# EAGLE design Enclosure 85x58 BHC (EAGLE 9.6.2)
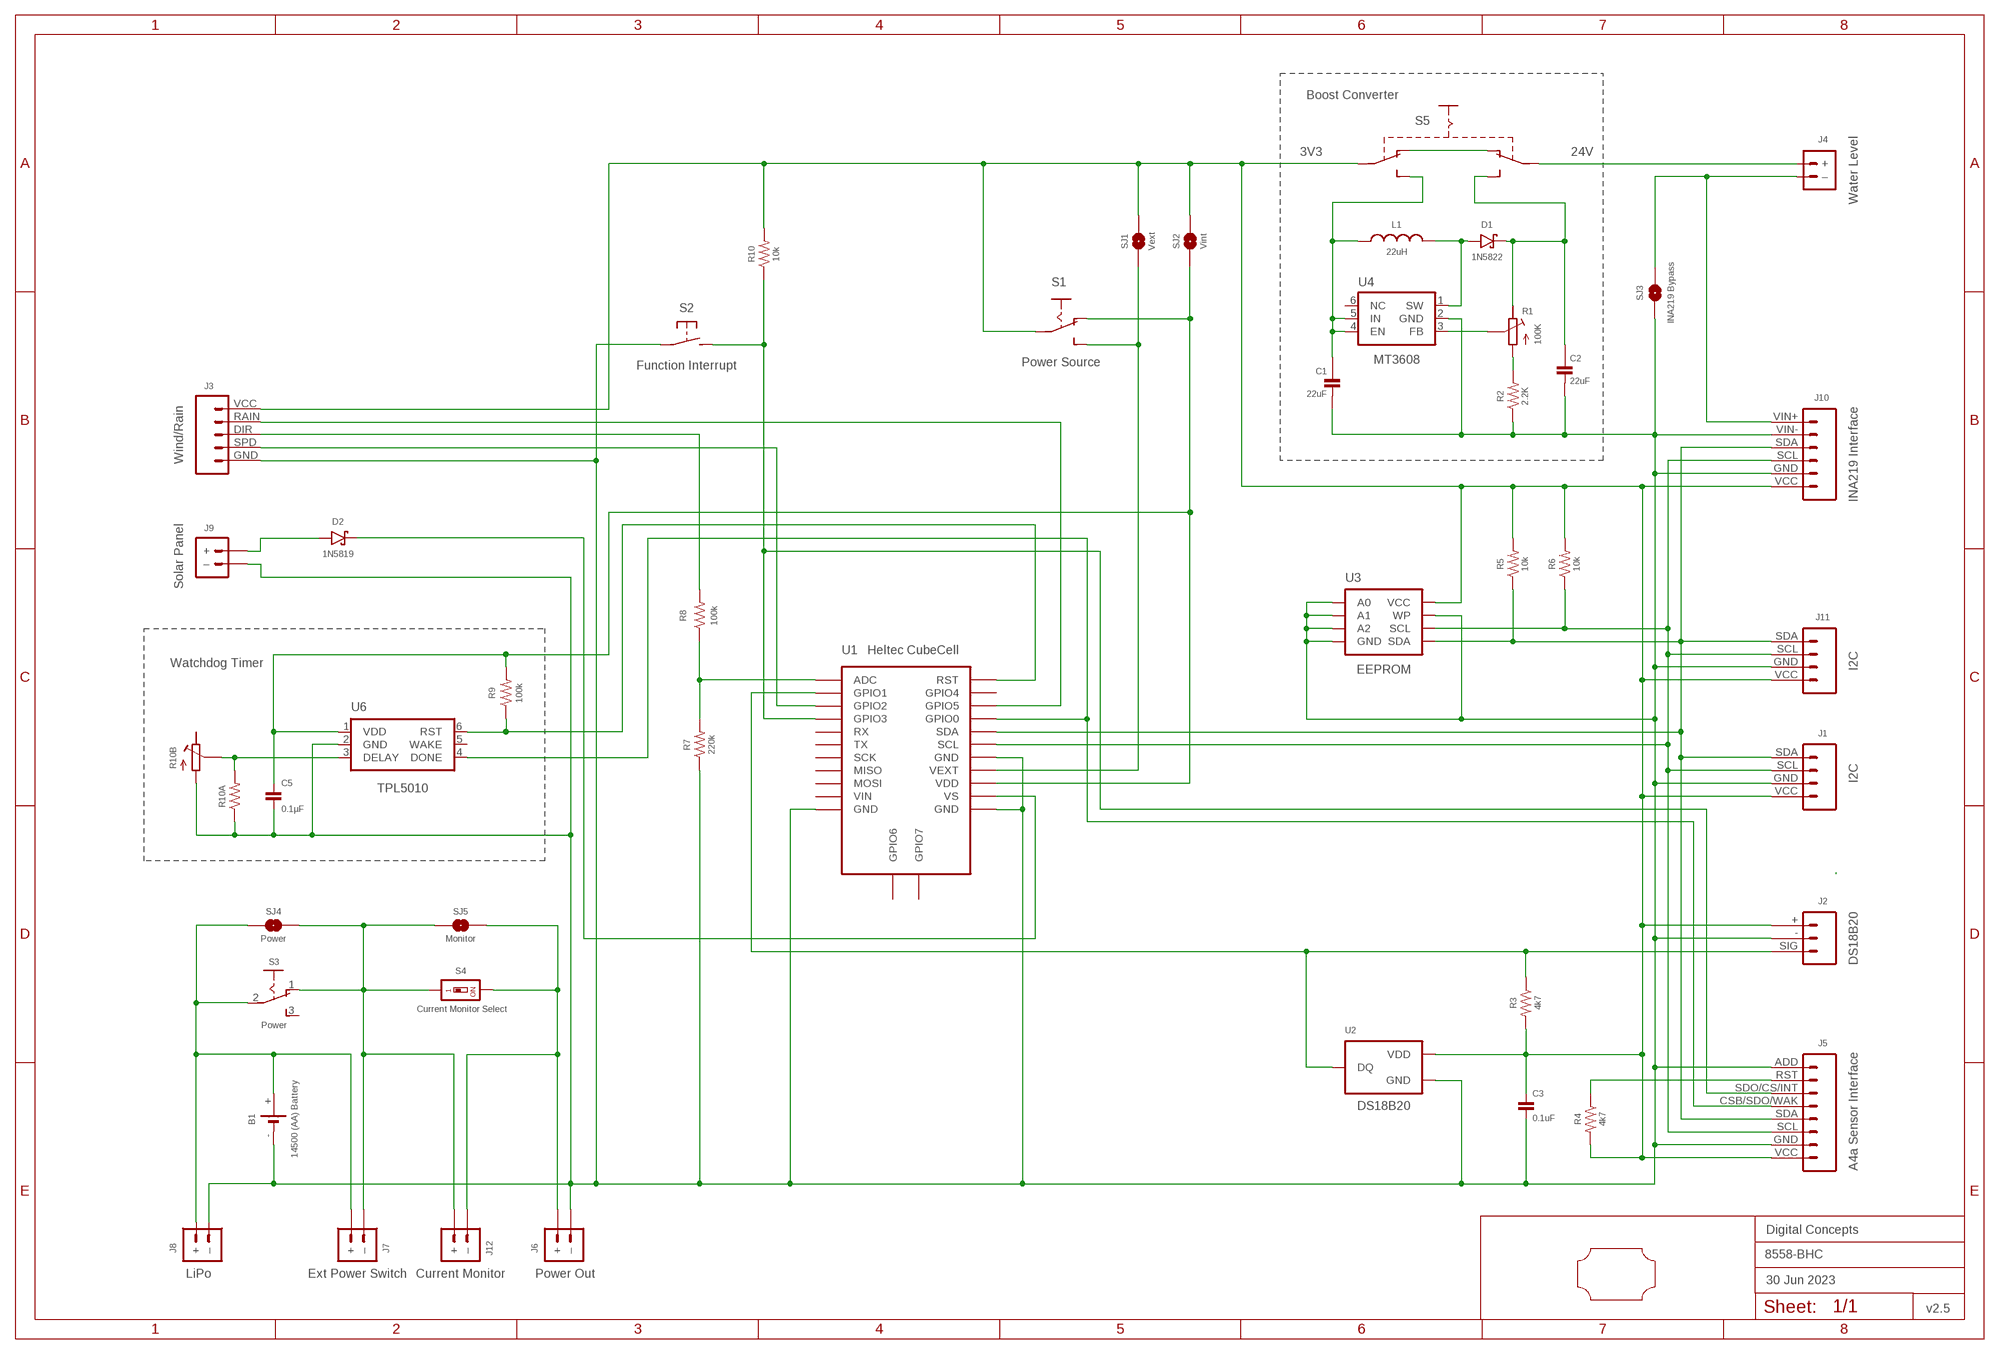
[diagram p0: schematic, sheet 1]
FRAME2 (A3L-LOC): DATE: 30 Jun 2023; OWNER: Digital Concepts; TITLE: 8558-BHC; VERSION: v2.5

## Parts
B1  14500 (AA) Battery  BATTERY-HOLDER-14500(AA)  [BATTERY-14500]
C1  22uF  CAPACITOR-1206  [C1206]
C2  22uF  CAPACITOR-1206  [C1206]
C3  0.1uF  CAPACITOR-0805  [C0805]
C5  0.1µF  CAPACITOR-0805  [C0805]
D1  1N5822  DIODE-SCHOTTKY-1N5822  [DIODE_SMB]
D2  1N5819  1N5819-SOD-123  [SOD-123]
J1  I2C  JST-PH2.0-4-VERTICAL-I2C  [JST-PH2.0-4-VERTICAL-I2C]
J2  DS18B20  JST-PH2.0-3-VERTICAL-DS18B20  [JST-PH2.0-3-VERTICAL]
J3  Wind/Rain  JST-PH2.0-5-VERTICAL-WEATHER  [JST-PH2.0-5-WEATHER]
J4  Water Level  JST-PH2.0-2-VERTICAL  [JST-PH2.0-2-VERTICAL=POWER]
J5  A4a Sensor Interface  HEADER-1X8-SENSOR  [CONN_08-SENSOR]
J6  Power Out  JST-GH1.25-2-HORIZONTAL-POWER  [JST-GH1.25-2-HORIZONTAL]
J7  Ext Power Switch  JST-PH2.0-2-DUAL-POWERJST-PTH-2  [JST-PH2.0-2-DUAL-POWER]
J8  LiPo  JST-PH2.0-2-MALE-HORIZONTALJST-PTH-2  [JST-PH2.0-2-HORIZONTAL]
J9  Solar Panel  JST-PH2.0-2-DUAL-POWERJST-PTH-2  [JST-PH2.0-2-DUAL-POWER]
J10  INA219 Interface  INA219-I2C-MODULE  [CONN_06-INA219]
J11  I2C  JST-PH2.0-4-HORIZONTAL-I2C  [JST-PH2.0-4-HORIZONTAL-I2C]
J12  Current Monitor  JST-PH2.0-2-HORIZONTAL-POWERJST-PTH-2  [JST-PH2.0-2-HORIZONTAL-POWER]
L1  22uH  INDUCTOR-CDRH104R/6D28L5038P  [CDRH104R+6D28]
R1  100K  RESISTOR-TRIMM-BAOTER-HORIZONTAL  [RTRIM64P]
R2  2.2K  RESISTORR0805  [R0805]
R3  4k7  RESISTORR0805  [R0805]
R4  4k7  RESISTORR0805  [R0805]
R5  10k  RESISTORR0805  [R0805]
R6  10k  RESISTORR0805  [R0805]
R7  220k  RESISTORR0805  [R0805]
R8  100k  RESISTORR0805  [R0805]
R9  100k  RESISTORR0805  [R0805]
R10  10k  RESISTORR0805  [R0805]
R10A  RESISTORR0805  [R0805]
R10B  RESISTOR-TRIMM-33  [RTRIM3*3]
S1  Power Source  SWITCH-SLIDE-SPDT-SMT  [SWITCH-SPDT-SMT]
S2  Function Interrupt  SWITCH-MOMENTARY-2-PIN  [SWITCH-2-PAD]
S3  Power  SWITCH-SLIDE-SPDT  [SWITCH-SLIDE-SPDT]
S4  Current Monitor Select  SWITCH-DIP-SWS001  [SMD-001]
S5  SWITCH-SLIDE-DPDT-PTH-S  [SWITCH-DPDT-PTH]
SJ1  Vext  SJ  [SJ]
SJ2  Vint  SJ-V-1  [SJ-VIA-1]
SJ3  INA219 Bypass  SJ  [SJ]
SJ4  Power  SJ  [SJ]
SJ5  Monitor  SJ  [SJ]
U1  Heltec CubeCell  HELTEC-CUBECELL  [HELTEC-CUBECELL]
U2  DS18B20  THERMOMETER-DS18B20  [TO-92]
U3  EEPROM  AT24CXX-EEPROM  [SOP-8]
U4  MT3608  [SOT-23-6@1]
U6  TPL5010  TPL5010DDCR  [SOT-23-6]
U$1  PCB-OUTLINE-C-85X58  [PROTO-28X18-OUTLINE-C]

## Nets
GND: B1.- C1.2 C2.2 C3.2 C5.2 J1.GND J2.- J3.GND J5.ADD J5.GND J6.-(–) J8.-(–) J9.-(–) J10.GND J10.VIN- J11.GND R2.1 R7.1 R10A.1 R10B.1(A) S2.P$1(P) SJ3.1 U1.GND@11(GND) U1.GND@14(GND) U1.GND@18(GND) U2.1(GND) U3.P$1(A0) U3.P$2(A1) U3.P$3(A2) U3.P$4(GND) U3.P$7(WP) U4.2(GND) U6.2(GND)
N$1: D2.A J9.+
N$2: J3.DIR R8.2
N$4: B1.+ J7.+ J8.+ S3.2(P) SJ4.2
N$5: D2.C U1.VS
N$6: D1.A L1.1 U4.1(SW)
N$7: C5.1 R9.2 S1.P$1(O) SJ2.2 U1.VDD U6.1(VDD)
N$8: J1.SCL J5.SCL J10.SCL J11.SCL R6.1 U1.SCL U3.P$6(SCL)
N$9: J5.RST R4.1
N$10: R7.2 R8.1 U1.ADC
N$11: J1.SDA J5.SDA J10.SDA J11.SDA R5.1 U1.SDA U3.P$5(SDA)
N$12: J3.SPD U1.GPIO2
N$14: J6.+ J12.-(–) S4.2 SJ5.1
N$15: J4.-(–) J10.VIN+ SJ3.2
N$18: J2.SIG R3.1 U1.GPIO1 U2.2(DQ)
N$19: J5.SDO/CS/INT R10.1 S2.P$2(S) U1.GPIO3
N$20: C2.1 D1.C R1.3(E) S5.P$3(S1)
N$21: S1.P$2(S) SJ1.2 U1.VEXT
N$22: J3.RAIN U1.GPIO5
N$23: R1.1(A) R2.2
N$24: R1.2(S) U4.3(FB)
N$25: C1.1 L1.2 S5.P$6(S2) U4.4(EN) U4.5(IN)
N$26: S5.P$1(O1) S5.P$4(O2)
N$27: J4.+ S5.P$2(P1)
N$28: J5.CSB/SDO/WAK U1.GPIO0 U6.4(DONE)
N$36: R10A.2 R10B.2(S) U6.3(DELAY)
N$37: R9.1 U1.RST U6.6(RST)
N$39: J7.-(–) J12.+ S3.1(O) S4.1 SJ4.1 SJ5.2
VCC: C3.1 J1.VCC J2.+ J3.VCC J5.VCC J10.VCC J11.VCC R3.2 R4.2 R5.2 R6.2 R10.2 S1.COMMON(P) S5.P$5(P2) SJ1.1 SJ2.1 SJ2.1@V U2.3(VDD) U3.P$8(VCC)
Unconnected: R10B.3(E) S3.3(S) U1.GPIO4 U1.GPIO6 U1.GPIO7 U1.MISO U1.MOSI U1.RX U1.SCK U1.TX U1.VIN U4.6(NC) U6.5(WAKE)

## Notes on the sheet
- Boost Converter
- 3V3 | 24V
- Watchdog Timer

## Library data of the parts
B1 = digitalconcepts:BATTERY-HOLDER-14500(AA): 14500 (AA) battery holder
C1 C2 = digitalconcepts:CAPACITOR-1206: 1206 Capacitor
C3 C5 = digitalconcepts:CAPACITOR-0805: 0805 Capacitor
D1 = digitalconcepts:DIODE-SCHOTTKY-1N5822: 1N5822 Schottky Diode SMB
D2 = digitalconcepts:1N5819-SOD-123: 1N5819 Schottky Diode SOD-123
J1 = digitalconcepts:JST-PH2.0-4-VERTICAL-I2C: PH2.0 4P I2C Vertical Connector
J2 = digitalconcepts:JST-PH2.0-3-VERTICAL-DS18B20: DS18B20 PH2.0 Vertical PCB Connector
J3 = digitalconcepts:JST-PH2.0-5-VERTICAL-WEATHER: PH2.0 5P Vertical Weather Connector
J4 = digitalconcepts:JST-PH2.0-2-VERTICAL: PH2.0 2P PCB Connector
J5 = digitalconcepts:HEADER-1X8-SENSOR: IoT Sensors 1x8 Pin Header for 'Sandwich' IoT Sensors
J6 = digitalconcepts:JST-GH1.25-2-HORIZONTAL-POWER: JST GH1.25 2P PTH Connector (Power)
J7 J9 = digitalconcepts:JST-PH2.0-2-DUAL-POWER: JST PH2.0 2P PTH Dual-Side Connector (Power); PROD_ID: CONN-09863; SKU: PRT-09914
J8 = digitalconcepts:JST-PH2.0-2-MALE-HORIZONTAL: PH2.0 2P Right Angle PCB Connector; PROD_ID: CONN-09863; SKU: PRT-09914
J10 = digitalconcepts:INA219-I2C-MODULE: INA219 I2C Module
J11 = digitalconcepts:JST-PH2.0-4-HORIZONTAL-I2C: PH2.0 4P I2C Horizontal Connector
J12 = digitalconcepts:JST-PH2.0-2-HORIZONTAL-POWER: PH2.0 2P Right Angle PCB Connector; PROD_ID: CONN-09863; SKU: PRT-09914
L1 = digitalconcepts:INDUCTOR-CDRH104R/6D28: Inductor; SPICEPREFIX: L
R1 = digitalconcepts:RESISTOR-TRIMM-BAOTER-HORIZONTAL: Trimm Resistor - Horizontal BAOTER
R2-R10 R10A = digitalconcepts:RESISTOR: Resistor; SPICEPREFIX: R
R10B = digitalconcepts:RESISTOR-TRIMM-3*3: Trimm Resistor - 3*3 SMD
S1 = digitalconcepts:SWITCH-SLIDE-SPDT-SMT: Mini Sliding Switch SPDT SMT
S2 = digitalconcepts:SWITCH-MOMENTARY-2-PIN: 2 Pin Momentary Switch
S3 = digitalconcepts:SWITCH-SLIDE-SPDT: Mini Sliding Switch SPDT
S4 = digitalconcepts:SWITCH-DIP-SWS001: SMD Dip Switch 1 pol.
S5 = digitalconcepts:SWITCH-SLIDE-DPDT-PTH-S: Switch DPDT PTH-S
SJ1 SJ3-SJ5 = digitalconcepts:SJ: Solder Jumper
SJ2 = digitalconcepts:SJ-V-1: Solder Jumper with single Pad Via
U1 = digitalconcepts:HELTEC-CUBECELL: Heltec CubeCell Development Board
U2 = digitalconcepts:THERMOMETER-DS18B20: Digital Thermometer -55C-125C TO92-3; AVAILABILITY: Bad; DESCRIPTION: Temperature Sensor Digital, Local -55°C ~ 125°C 12 b 8-uMAX; MF: Maxim Integrated; MP: DS18B20; PACKAGE: TO-92 Maxim Integrated; PRICE: None
U3 = digitalconcepts:AT24CXX-EEPROM: AT24Cxx EEPROM SOP-8
U4 = digitalconcepts:MT3608: MT3608 DC-DC Step-Up Voltage Converter
U6 = digitalconcepts:TPL5010DDCR: TPL5010 Nano-Power System Timer with Watchdog
U$1 = digitalconcepts:PCB-OUTLINE-C-85X58: PCB outline with cut-out for 85 x 58 enclosure

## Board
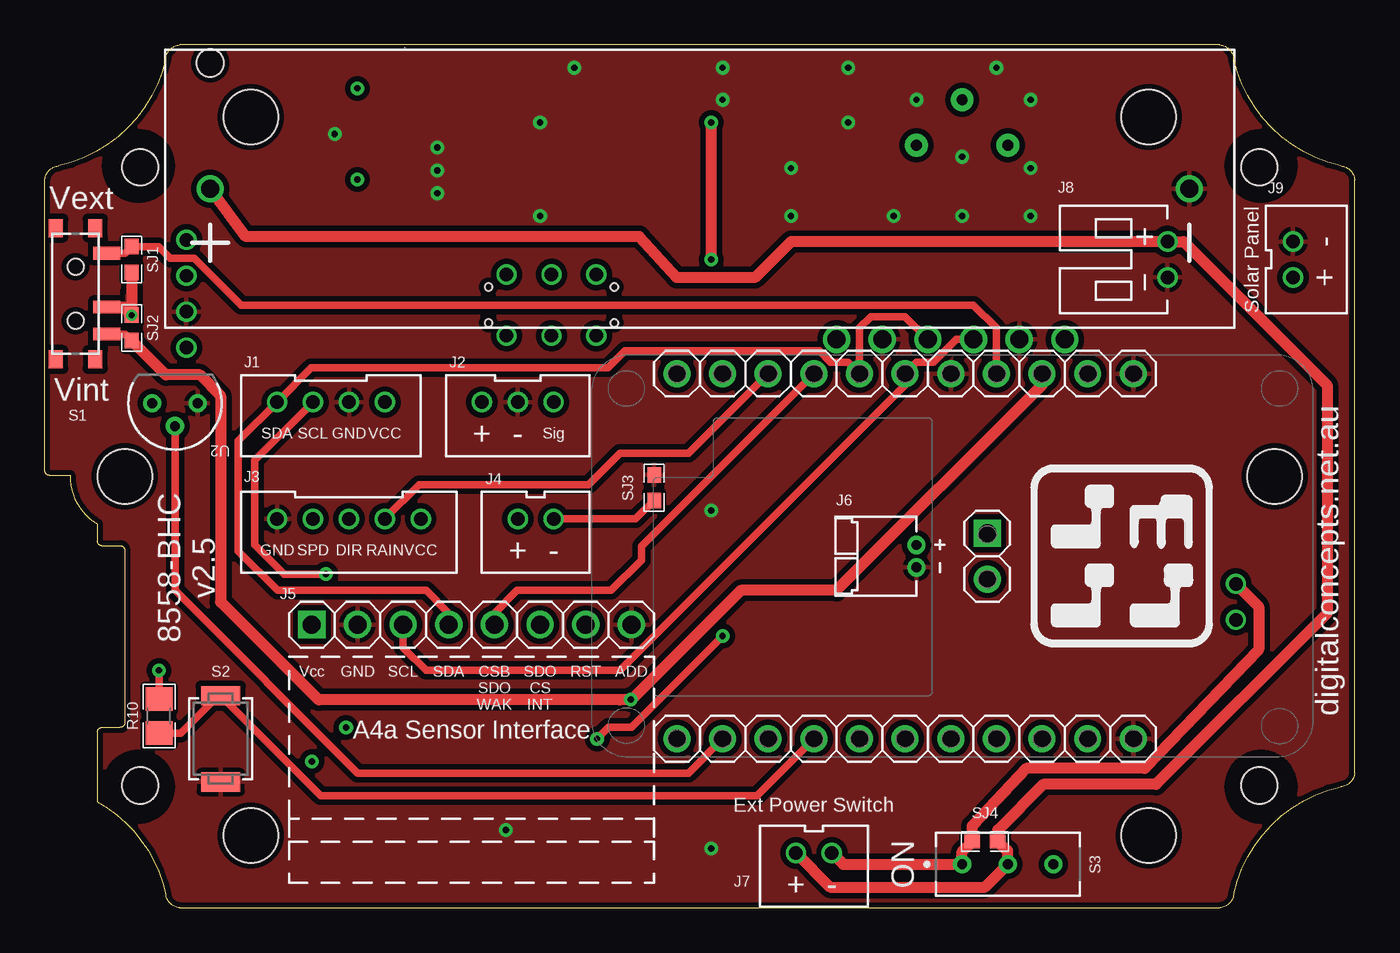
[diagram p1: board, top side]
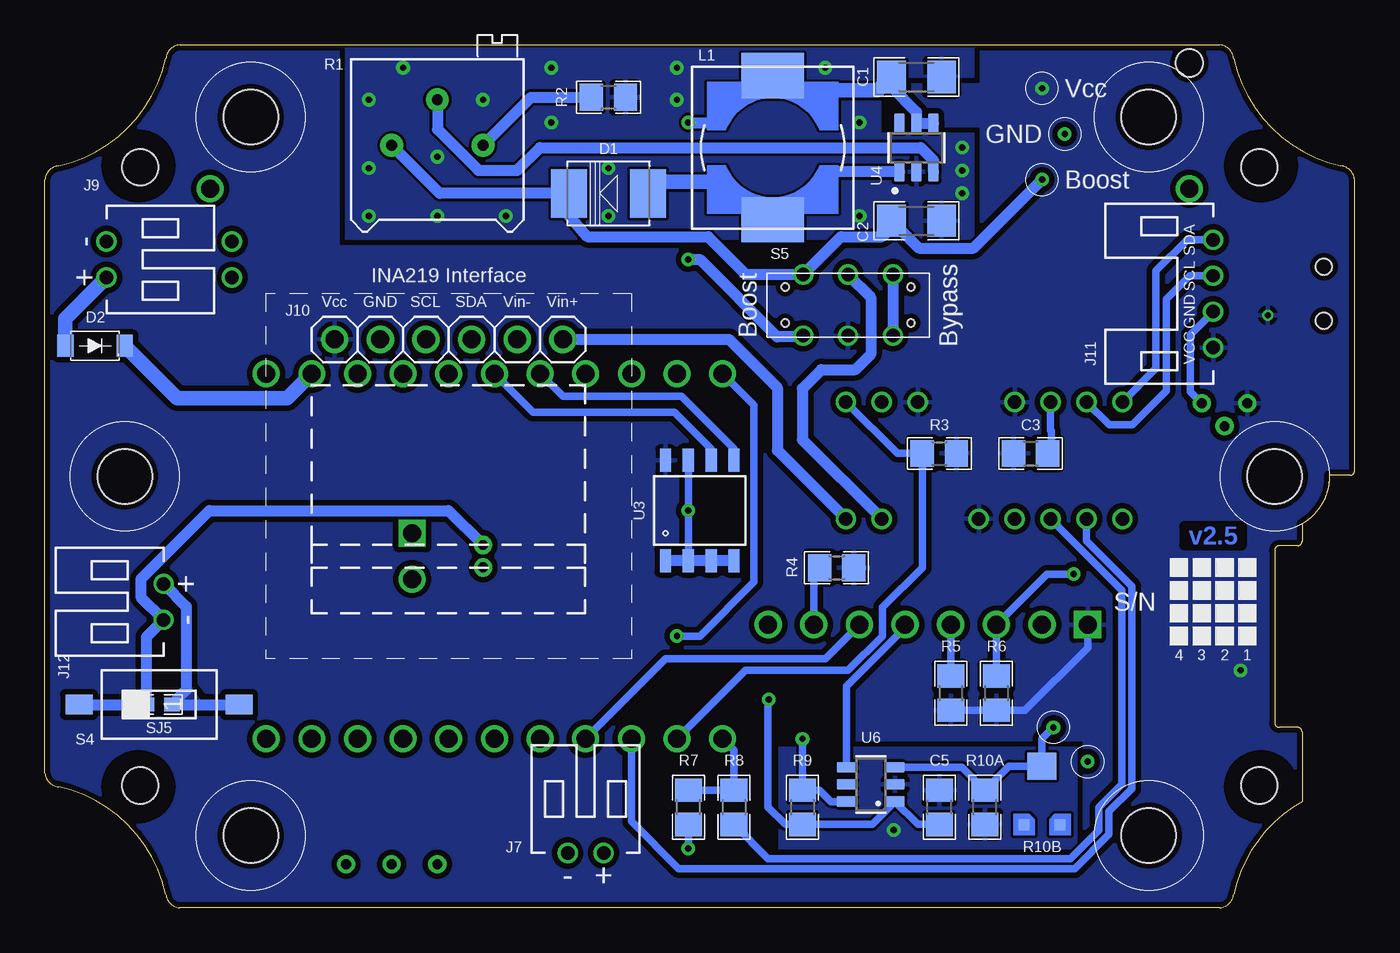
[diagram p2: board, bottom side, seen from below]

Size 72.9 x 48.01 mm. Coordinates in mm from the lower left corner, seen from the top.
Copper layers (1*16): Top 0.035mm / dielectric 1.5mm / Bottom 0.035mm
Design rules "default *": minimum track width 6mil, minimum drill 0.35mm, track to track 6mil, track to pad 6mil, pad to pad 6mil, via to via 6mil, smd to smd 6mil, copper to edge 6mil, drill to drill 6mil, minimum pad ring 1mil, minimum via ring 8mil, stop-mask expansion 4mil, vias tented up to drill 0mil, thermal gap 10mil

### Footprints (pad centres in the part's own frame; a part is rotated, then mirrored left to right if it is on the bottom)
BATTERY-14500 = drill 1: + -27.25,0; - 27.25,0 | hole 1.524: -27.25,7
C1206 = smd 1.6 x 1.8: 1 -1.4,0; 2 1.4,0
C0805 = smd 1.3 x 1.5: 1 -0.95,0; 2 0.95,0
DIODE_SMB = smd 2 x 2.7: A 2.2,0; C -2.2,0
SOD-123 = smd 0.91 x 1.22: A -1.65,0; C 1.65,0
JST-PH2.0-4-VERTICAL-I2C = drill 0.75: GND 1,0; SCL -1,0; SDA -3,0; VCC 3,0
JST-PH2.0-3-VERTICAL = drill 0.75: + -2,0; - 0,0; SIG 2,0
JST-PH2.0-5-WEATHER = drill 0.75: DIR 0,0; GND 4,0; RAIN -2,0; SPD 2,0; VCC -4,0
JST-PH2.0-2-VERTICAL=POWER = drill 0.75: + -1,0; - 1,0
CONN_08-SENSOR = drill 1 pad 1.524: ADD 17.78,0; CSB/SDO/WAK 10.16,0; GND 2.54,0; RST 15.24,0; SCL 5.08,0; SDA 7.62,0; SDO/CS/INT 12.7,0 | drill 1 pad 1.524 square: VCC 0,0
JST-GH1.25-2-HORIZONTAL = drill 0.55 pad 1.016: + -0.625,0; - 0.625,0
JST-PH2.0-2-DUAL-POWER = drill 0.75: + 1,0; - -1,0
JST-PH2.0-2-HORIZONTAL = drill 0.75: + 1,0; - -1,0
CONN_06-INA219 = drill 1 pad 1.524: GND 2.54,0; SCL 5.08,0; SDA 7.62,0; VCC 0,0; VIN+ 12.7,0; VIN- 10.16,0
JST-PH2.0-4-HORIZONTAL-I2C = drill 0.75: GND -1,0; SCL 1,0; SDA 3,0; VCC -3,0
JST-PH2.0-2-HORIZONTAL-POWER = drill 0.75: + 1,0; - -1,0
CDRH104R+6D28 = smd 2.5 x 3.5: 1 -4,0; 2 4,0
RTRIM64P = drill 0.61 pad 1.27: 1 0,-2.54; 2 2.54,0; 3 0,2.54
R0805 = smd 1.3 x 1.5: 1 -0.95,0; 2 0.95,0
RTRIM3*3 = smd 0.6 x 0.6: 1 -1,-1.6; 3 1,-1.6 | smd 1.6 x 1.5: 2 0,1.65
SWITCH-SPDT-SMT = smd 0.7 x 1.5: COMMON 0.75,1.75; P$1 2.25,1.75; P$2 -2.25,1.75 | smd 1 x 0.8: GND@1 3.65,-1.1; GND@2 3.65,1.1; GND@3 -3.65,1.1; GND@4 -3.65,-1.1 | hole 0.9: -1.5,0; 1.5,0
SWITCH-2-PAD = smd 1.067 x 2.184: P$1 -2.4,0; P$2 2.4,0
SWITCH-SLIDE-SPDT = drill 0.55 pad 1.016: 1 -2.54,0; 2 0,0; 3 2.54,0
SMD-001 = smd 1.1 x 1.5: 1 0,-4.45; 2 0,4.45
SWITCH-DPDT-PTH = drill 0.75: P$1 -1.7,2.5; P$2 -1.7,0; P$3 -1.7,-2.5; P$4 1.7,2.5; P$5 1.7,0; P$6 1.7,-2.5 | hole 0.42: 1,3.5; -1,3.5; 1,-3.5; -1,-3.5
SJ = smd 0.864 x 0.762: 1 -0.711,0; 2 0.711,0
SJ-VIA-1 = smd 0.864 x 0.762: 1 -0.711,0; 2 0.711,0 | drill 0.35 pad 0.61: 1@V -0.711,0
HELTEC-CUBECELL = drill 1: ADC 0,0; GND@11 0,25.4; GND@14 -20.32,25.4; GND@18 -20.32,15.24; GPIO0 -20.32,7.62; GPIO1 0,2.54; GPIO2 0,5.08; GPIO3 0,7.62; GPIO4 -20.32,2.54; GPIO5 -20.32,5.08; GPIO6 -8.89,17.272; MISO 0,17.78; MOSI 0,20.32; RST -20.32,0; RX 0,10.16; SCK 0,15.24; SCL -20.32,12.7; SDA -20.32,10.16; TX 0,12.7; VDD -20.32,20.32; VEXT -20.32,17.78; VIN 0,22.86; VS -20.32,22.86 | drill 1 square: GPIO7 -11.43,17.272
TO-92 = drill 0.55 pad 1.016: 1 -1.27,0; 2 0,1.27; 3 1.27,0
SOP-8 = smd 0.635 x 1.27: P$1 -1.905,-2.794; P$2 -0.635,-2.794; P$3 0.635,-2.794; P$4 1.905,-2.794; P$5 1.905,2.794; P$6 0.635,2.794; P$7 -0.635,2.794; P$8 -1.905,2.794
SOT-23-6@1 = smd 1.1 x 0.6: 1 -1.35,0.95; 2 -1.35,0; 3 -1.35,-0.95; 4 1.35,-0.95; 5 1.35,0; 6 1.35,0.95
SOT-23-6 = smd 1.1 x 0.6: 1 -1.35,0.95; 2 -1.35,0; 3 -1.35,-0.95; 4 1.35,-0.95; 5 1.35,0; 6 1.35,0.95
PROTO-28X18-OUTLINE-C = hole 2.032: -31.14,17.196; -31.14,-17.196; 31.14,-17.196; 31.14,17.196 | hole 3.048: -24.994,19.99; -32.004,0; -24.994,-19.99; 24.994,-19.99; 32.004,0; 24.994,19.99

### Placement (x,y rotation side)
B1  36.45,40.01 0 top
C1  24.38,46.23 0 bottom
C2  24.38,38.23 0 bottom
C3  18.03,25.27 0 bottom
C5  23.11,5.59 90 bottom
D1  41.53,39.75 0 bottom
D2  70.1,31.27 0 bottom
J1  15.92,28.13 0 top
J2  26.32,28.13 0 top
J3  16.92,21.63 180 top
J4  27.32,21.63 0 top
J5  14.86,15.75 0 top
J6  48.51,19.56 270 top
J7  42.8,3.05 0 bottom
J8  62.48,36.07 90 top
J9  69.47,36.07 270 bottom
J10  56.77,31.62 0 bottom
J11  7.87,34.16 90 bottom
J12  66.29,17.02 90 bottom
L1  32.38,42.29 90 bottom
R1  51.05,42.42 90 bottom
R2  41.53,45.09 180 bottom
R3  23.11,25.27 0 bottom
R4  28.83,18.92 0 bottom
R5  22.48,11.94 270 bottom
R6  19.94,11.94 270 bottom
R7  37.08,5.59 90 bottom
R8  34.54,5.59 270 bottom
R9  30.73,5.59 270 bottom
R10  6.35,10.67 90 top
R10A  20.57,5.59 90 bottom
R10B  17.4,6.22 0 bottom
S1  1.7,34.16 270 top
S2  9.78,9.4 90 top
S3  53.59,2.41 0 top
S4  66.55,11.3 90 bottom
S5  28.19,33.53 270 bottom
SJ1  4.83,36.07 90 top
SJ2  4.83,32.26 270 top
SJ3  33.91,23.37 270 top
SJ4  52.32,3.68 0 top
SJ5  66.55,11.3 0 bottom
U1  35.18,9.4 270 top
U2  7.24,28.07 180 top
U3  36.45,22.1 0 bottom
U4  24.38,42.29 90 bottom
U6  26.92,6.86 180 bottom
U$1  36.45,24 0 top

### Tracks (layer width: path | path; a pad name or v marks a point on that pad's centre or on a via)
$X1
  cutout Bottom: 67.69,43.31 arc180 67.69,39.24 arc180
$X2
  cutout Bottom: 67.69,8.76 arc180 67.69,4.7 arc180
$X3
  cutout Bottom: 5.21,8.76 arc180 5.21,4.7 arc180
$X4
  cutout Bottom: 5.21,43.31 arc180 5.21,39.24 arc180
$X5
  cutout Top: 5.21,43.31 arc180 5.21,39.24 arc180
$X6
  cutout Top: 67.69,43.31 arc180 67.69,39.24 arc180
$X7
  cutout Top: 67.69,8.76 arc180 67.69,4.7 arc180
$X8
  cutout Top: 5.21,8.76 arc180 5.21,4.7 arc180
GND  (via drill 0.35)
  Bottom 0.406: C3.2 16.89,25.47 16.89,26.54 16.92,26.57 J1.GND | R7.1 v37.08,3.3 | U3.P$7 v37.08,22.1 U3.P$2 | J11.GND 9.14,31.89 9.14,28.7 U2.1
  Bottom 0.61: U3.P$4 U3.P$3 U3.P$2 U3.P$1
  other vias: 21.84,42.29 27.56,43.69 37.72,44.96 37.72,46.74 44.7,46.74 44.7,43.69 41.53,38.48 47.24,38.48 51.05,38.48 51.05,41.78 54.86,38.48 54.86,41.15 52.96,46.74 21.84,39.75 48.51,44.96 54.86,44.96 27.56,38.48 41.53,41.15 16.13,43.05 21.84,41.02 29.46,46.74 25.65,4.32
  pour Top (isolate 0.305, rank 2): -2.08,49.93 -2.08,-1.97 74.92,-1.97 74.92,49.93
  pour Bottom (rank 2): 21.21,48.13 21.21,46.23 26.42,46.23 26.42,43.05 21.21,43.05 21.21,37.21 56.13,37.21 56.13,48.13
  pour Bottom: 32,8.89 15.49,8.89 15.49,3.3 32,3.3
GND1  (via drill 0.35)
  other vias: 14.86,8.13
N$1
  Bottom 0.813: J9.+ 71.75,32.78 D2.A
N$2
  Bottom 0.406: J3.DIR 12.95,17.67 12.95,6.86 14.22,5.59 14.22,4.32 15.81,2.73 32.64,2.73 R8.2
N$4
  Top 0.61: B1.+ 11.18,37.34 33.09,37.34 35.18,35.05 39.51,35.05 41.53,37.07 J8.+ 63.39,37.07 71.37,29.08 71.37,16.38 61.85,6.86 55.58,6.86 53.03,4.32 SJ4.2 53.52,3.19 53.59,3.18 S3.2 52.32,1.14 43.7,1.14 J7.+
N$5
  Bottom 0.813: D2.C 65.53,28.35 59.41,28.35 U1.VS
N$6
  Bottom 0.61: L1.1 31.75,38.29 29.1,40.94 U4.1
  Bottom 0.813: D1.A 38.69,40.39 35.17,40.39 33.08,38.29 L1.1
N$7  (via drill 0.35)
  Top 0.406: SJ2.2 4.46,31.91 S1.P$1
  Top 0.61: 32.59,11.56 32.64,11.56 38.73,17.65 44.07,17.65 55.5,29.08 U1.VDD | SJ2.2 6.73,29.64 8.64,29.64 9.78,28.5 9.78,17.02 15.24,11.56 32,11.56 32.59,11.56 | v32.61,11.58 32.59,11.56
  Bottom 0.406: C5.1 24.3,4.64 U6.1 26.84,4.64 R9.2 31.69,4.64 32.64,5.59 32.64,11.56 v32.61,11.58
N$8  (via drill 0.35)
  Top 0.406: J5.SCL 19.94,14.48 21.21,13.21 32,13.21 47.88,29.08 U1.SCL 48.51,30.35 49.47,30.35 50.74,31.62 J10.SCL | v15.64,18.57 13.31,18.57 11.68,20.19 11.68,24.9 J1.SCL
  Bottom 0.406: v15.64,18.57 17.12,18.57 J5.SCL R6.1 | U3.P$6 35.81,25.53 37.85,27.56 45.72,27.56 U1.SCL | J11.SCL 9.16,35.16 10.47,33.85 10.47,28.77 12.38,26.86 13.65,26.86 J1.SCL
N$9
  Bottom 0.406: R4.1 30.1,18.6 J5.RST
N$10
  Bottom 0.406: R7.2 R8.1 34.54,8.76 U1.ADC
N$11
  Top 0.406: J10.SDA 47.88,32.89 45.97,32.89 45.34,32.26 U1.SDA 44.7,30.35 43.74,30.35 43.1,30.99 32.28,30.99 31.33,30.04 14.82,30.04 J1.SDA 10.77,25.98 10.77,19.84 12.95,17.65 21.21,17.65 22.48,16.38 J5.SDA
  Bottom 0.406: J11.SDA 9.32,37.16 11.05,35.43 11.05,30 J1.SDA | U1.SDA 44.07,28.45 37.46,28.45 34.54,25.53 U3.P$5 | J5.SDA R5.1
N$12
  Bottom 0.406: J3.SPD 14.92,20.42 12.39,17.9 12.39,6.63 13.66,5.36 13.66,4.09 15.58,2.17 37.63,2.17 40.26,4.8 U1.GPIO2
N$14
  Bottom 0.61: S4.2 SJ5.1 67.26,15.05 J12.- 67.56,17.29 67.56,18.29 63.75,22.1 50.43,22.1 J6.+
N$15
  Top 0.406: J4.- 32.88,21.63 SJ3.2
  Bottom 0.61: J4.- 32.13,25.44 32.13,28.94 34.81,31.62 J10.VIN+
N$18
  Top 0.406: U1.GPIO1 35.81,7.49 17.4,7.49 7.24,17.65 U2.2
  Bottom 0.406: J2.SIG 25.46,25.27 R3.1 24.06,18.93 26.29,16.71 26.29,15.11 28.19,13.21 33.91,13.21 U1.GPIO1
N$19
  Top 0.406: R10.1 7.56,9.72 9.64,11.8 S2.P$2 15.35,6.22 39.62,6.22 U1.GPIO3
  Bottom 0.406: U1.GPIO3 38.35,13.84 29.46,13.84 J5.SDO/CS/INT
N$20  (via drill 0.35)
  Bottom 0.61: v17.4,40.51 21.21,36.7 24.26,36.7 C2.1 25.78,37.84 26.29,37.34 28.58,37.34 S5.P$3 33.87,35.23 35.98,37.34 42.71,37.34 43.73,38.51 D1.C 50.93,39.75 R1.3
N$21
  Top 0.406: U1.VEXT 52.96,32.26 51.69,33.53 10.92,33.53 8.31,36.14 6.96,36.14 6.34,36.78 SJ1.2 4.46,36.41 S1.P$2
N$22
  Top 0.406: J3.RAIN 20.82,23.54 30.27,23.54 32,25.27 35.81,25.27 U1.GPIO5
N$23
  Bottom 0.61: R1.1 45.85,45.09 R2.2
N$24
  Bottom 0.61: R1.2 51.05,43.31 48.77,41.02 46.61,41.02 45.34,42.29 24.15,42.29 23.43,41.58 U4.3
N$25  (via drill 0.35)
  Top 0.61: v37.08,43.69 v37.08,36.07
  Bottom 0.61: C1.1 25.78,45.67 24.38,44.27 U4.5 U4.4 | v37.08,43.69 35.81,43.69 33.21,46.29 L1.2 | 30.69,31.76 32.14,31.76 36.45,36.07 v37.08,36.07
  Bottom 0.813: C1.1 26.53,45.48 31.58,45.48 L1.2 | S5.P$6 30.69,31.76
N$26
  Bottom 0.61: S5.P$1 S5.P$4
N$27
  Bottom 0.61: J4.+ 30.73,26.05 30.73,28.88 29.68,29.93 27.77,29.93 26.92,30.78 26.92,33.96 S5.P$2
N$28
  Top 0.406: U1.GPIO0 33.2,20.12 33.2,19.33 31.52,17.65 26.29,17.65 25.02,16.38 J5.CSB/SDO/WAK
  Bottom 0.406: J5.CSB/SDO/WAK 25.02,15.59 28.27,12.33 U6.4
N$36  (via drill 0.35)
  Bottom 0.406: U6.3 21.84,7.81 R10A.2 19.24,7.87 R10B.2 17.4,9.4 v16.76,10.03
N$37  (via drill 0.35)
  Top 0.406: v30.73,9.4 31.37,10.03 32.64,10.03 v37.72,15.11
  Bottom 0.406: U6.6 29.15,5.91 29.78,6.54 R9.1 v30.73,9.4 | U1.RST 33.42,27.96 33.42,18.14 36.45,15.11 v37.72,15.11
N$39
  Top 0.61: J12.+ 67.56,16.75 67.56,14.35 61.21,7.75 54.62,7.75 51.61,4.55 SJ4.1 51.05,3.12 S3.1 44.43,2.41 J7.-
  Bottom 0.61: J12.+ 65.02,16.75 65.02,12.12 SJ5.2 S4.1
  pour Bottom: 65.85,11.3 65.02,12.12 64.39,11.3
VCC  (via drill 0.35)
  Top 0.406: R10.2 v6.35,13.21
  Top 0.61: S1.COMMON 4.38,33.41 SJ2.1@V SJ1.1
  Bottom 0.406: R5.2 R6.2 18.35,10.99 14.86,14.48 J5.VCC
  other vias: 17.4,45.59
  pour Bottom (isolate 0.305, rank 5): -1.08,48.93 -1.08,-0.97 73.92,-0.97 73.92,48.93
  pour Top: 4.22,33.46 4.7,33.93 4.7,32.98

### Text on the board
Bottom: v2.5
tPlace: digitalconcepts.net.au | 8558-BHC / v2.5
bPlace: Vin+ | Vin- | SDA | SCL | GND | Vcc | S/N | 1 | 2 | 3 | 4
tNames: Vext | Solar Panel | Vint | Vcc | GND | SCL | SDA | RST | ADD | CSB / SDO / WAK | SDO / CS / INT | ON
bNames: Vcc | GND | Boost | J9 | Bypass | Boost | J7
